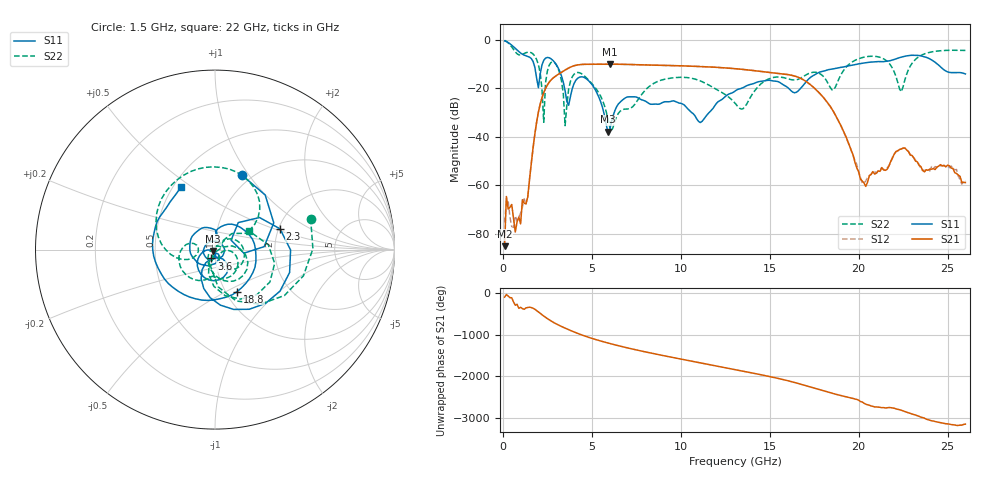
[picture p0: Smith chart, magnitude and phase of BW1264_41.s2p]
!Keysight Technologies,N5245B,MY57181159,A.13.60.06
!Date: Friday, December 18, 2020 23:54:14
!Correction: S11(Full 2 Port(1,2))
!S21(Full 2 Port(1,2))
!S12(Full 2 Port(1,2))
!S22(Full 2 Port(1,2))
!S2P File: Measurements: S11, S21, S12, S22:
# Hz S  dB  R 50
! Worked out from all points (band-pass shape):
!   260 points, 100 MHz to 26 GHz, reference 50 ohm
!   highest |S21| = -9.99 dB at 6 GHz (marker M1); lowest = -85.1 dB at 100 MHz (marker M2)
!   |S21| within 3 dB of the highest: 3.371 GHz to 14.5 GHz (11.13 GHz wide, 125 % of centre)
!   lowest |S11| = -37.9 dB at 5.9 GHz (marker M3), VSWR 1.03, Z = 49 - j0.8 ohm
!   |S11| at or under -10 dB: 1.748 GHz to 2.216 GHz (468 MHz wide, 23.6 % of centre); 2.985 GHz to 19.92 GHz (16.93 GHz wide, 148 % of centre); 24.44 GHz to end of sweep
!   |S22| runs from -37.8 to -0.2 dB; largest |S21 - S12| = 0.00063
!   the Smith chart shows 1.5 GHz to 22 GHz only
!   S11 on the Smith chart (normalised r, x): 1.5 GHz: 0.89, +0.93; 2.3 GHz: 2.04, +0.55; 3.6 GHz: 0.95, -0.09; 18.8 GHz: 1.13, -0.57; 22 GHz: 0.55, +0.45
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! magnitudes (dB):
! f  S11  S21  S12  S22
! 100 MHz  -0.4  -85.1  -75.4  -0.2
! 200 MHz  -0.6  -64.6  -66.2  -0.6
! 700 MHz  -3.4  -79.3  -72.6  -4.9
! 1.5 GHz  -7.1  -57.7  -57.4  -5.0
! 2.1 GHz  -14.0  -26.5  -26.5  -13.6
! 2.3 GHz  -8.4  -21.7  -21.7  -34.0
! 2.7 GHz  -7.7  -16.6  -16.6  -9.3
! 3.3 GHz  -14.9  -13.3  -13.3  -17.0
! 3.5 GHz  -20.9  -12.4  -12.4  -35.4
! 3.6 GHz  -25.4  -12.0  -12.0  -26.8
! 4.5 GHz  -15.3  -10.1  -10.1  -14.3
! 5.9 GHz  -37.9  -10.0  -10.0  -32.3
! 6 GHz  -37.6  -10.0  -10.0  -35.7
! 8.8 GHz  -26.5  -10.4  -10.4  -16.8
! 11.1 GHz  -34.1  -11.0  -11.0  -16.9
! 13.1 GHz  -20.9  -11.9  -11.9  -26.5
! 17.4 GHz  -14.9  -19.2  -19.2  -13.4
! 18.8 GHz  -11.5  -32.5  -32.4  -17.6
! 20.2 GHz  -9.7  -58.3  -59.1  -7.3
! 21.7 GHz  -8.6  -52.1  -51.9  -9.5
! 22 GHz  -8.1  -47.1  -47.2  -13.2
! 26 GHz  -14.0  -58.9  -58.3  -4.3
